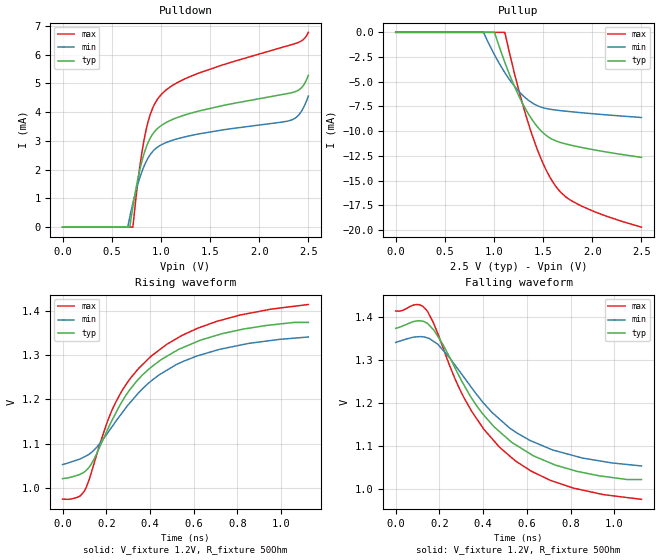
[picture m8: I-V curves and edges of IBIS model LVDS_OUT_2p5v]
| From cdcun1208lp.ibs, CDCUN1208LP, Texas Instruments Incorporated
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[Model]   LVDS_OUT_2p5v
Model_type   Output
Polarity   Non-Inverting
Enable   Active-High
Vmeas = 1.2
Vref = 1.2
Cref = 0pF
Rref = 50
|   typ   min   max
C_comp   6.0572pF   5.8048pF   6.5468pF
[Voltage Range]   2.5   2.375   2.625
[Temperature Range]   27   105   -40
[Pullup Reference]   2.5   2.375   2.625
[Pulldown Reference]   0   0   -0
[Power Clamp Reference]   2.5   2.375   2.625
[GND Clamp Reference]   0   0   0
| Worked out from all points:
|   falling waveform, V_fixture 1.2V, R_fixture 50Ohm: 20-80 % time 332ps typ, 345ps min, 335ps max; typ from 1.37 V to 1.02 V
|   rising waveform, V_fixture 1.2V, R_fixture 50Ohm: 20-80 % time 329ps typ, 355ps min, 335ps max; typ from 1.02 V to 1.37 V
[Pulldown]
|   Voltage   I(typ)   I(min)   I(max)
0V        0A         0A         0A
657.9mV   0A         0A         0A
683mV     0A         338uA      0A
714.3mV   693.3uA    823uA      0A
783.2mV   1.957mA    1.693mA    2.039mA
845.9mV   2.734mA    2.25mA     3.322mA
914.8mV   3.23mA     2.626mA    4.13mA
1.003V    3.533mA    2.862mA    4.61mA
1.372V    4.03mA     3.236mA    5.344mA
2.325V    4.675mA    3.724mA    6.346mA
2.419V    4.815mA    3.977mA    6.461mA
2.5V      5.283mA    4.562mA    6.781mA
[Pullup]
|   Voltage   I(typ)   I(min)   I(max)
0V        0A         0A         0A
889.7mV   0A         0A         0A
1.003V    0A         -2.225mA   0A
1.109V    -3.003mA   -4.056mA   0A
1.247V    -6.312mA   -5.902mA   -5.652mA
1.372V    -8.601mA   -7.028mA   -9.914mA
1.497V    -10.15mA   -7.62mA    -13.22mA
1.617V    -10.93mA   -7.846mA   -15.41mA
1.729V    -11.29mA   -7.976mA   -16.63mA
1.873V    -11.61mA   -8.115mA   -17.49mA
2.149V    -12.11mA   -8.351mA   -18.61mA
2.5V      -12.65mA   -8.613mA   -19.7mA
[Ramp]
R_load = 50
|   typ   min   max
dV/dt_r   0.21133/3.28578e-010  0.172601/3.54442e-010  0.263179/3.35251e-010
dV/dt_f   0.21133/3.32017e-010  0.172601/3.45016e-010  0.263179/3.34923e-010
[Falling Waveform]
V_fixture = 1.2V
V_fixture_min = 1.2V
V_fixture_max = 1.2V
R_fixture = 50Ohm
C_fixture = 0F
|   Time   V(typ)   V(min)   V(max)
0s        1.373V     1.341V     1.414V
97.64ps   1.391V     1.353V     1.429V
144.8ps   1.385V     1.351V     1.414V
193.1ps   1.354V     1.336V     1.361V
275.1ps   1.278V     1.285V     1.251V
348.6ps   1.21V      1.234V     1.179V
449.7ps   1.144V     1.173V     1.111V
547.7ps   1.103V     1.132V     1.065V
829.2ps   1.04V      1.075V     999.5mV
1.124ns   1.021V     1.053V     975.2mV
[Rising Waveform]
V_fixture = 1.2V
V_fixture_min = 1.2V
V_fixture_max = 1.2V
R_fixture = 50Ohm
C_fixture = 0F
|   Time   V(typ)   V(min)   V(max)
0s        1.021V     1.053V     975.2mV
99.33ps   1.036V     1.07V      993.1mV
146ps     1.067V     1.087V     1.058V
198.9ps   1.124V     1.119V     1.141V
243.4ps   1.169V     1.15V      1.194V
306.2ps   1.221V     1.191V     1.244V
404.2ps   1.272V     1.241V     1.297V
554.9ps   1.318V     1.286V     1.346V
729.6ps   1.348V     1.314V     1.379V
1.124ns   1.373V     1.341V     1.414V
